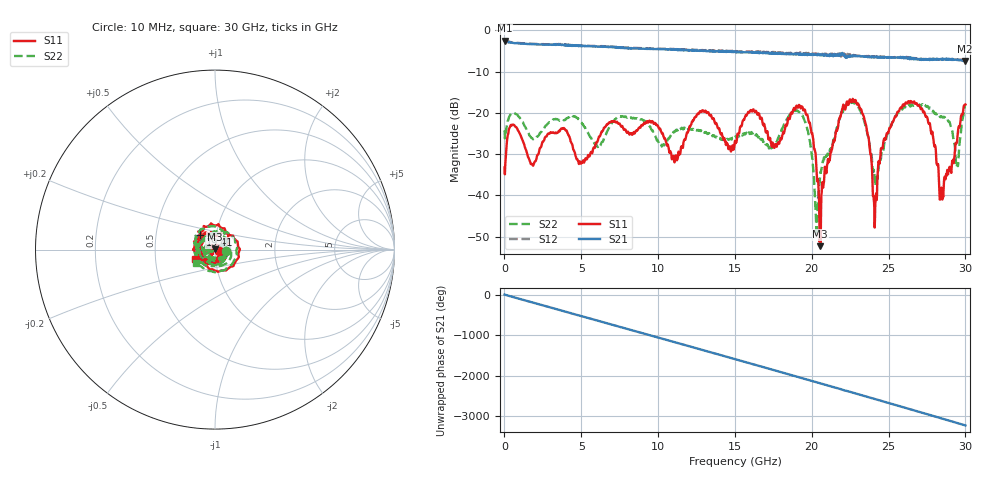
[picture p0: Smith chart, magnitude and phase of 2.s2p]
!Agilent Technologies,E8364B,US42250130,A.04.87.01
!Agilent E8364B: A.04.87.01
!Date: Monday, February 07, 2022 23:47:05
!Correction: S11(Full 2 Port SOLT,1,2) S21(Full 2 Port SOLT,1,2) S12(Full 2 Port SOLT,1,2) S22(Full 2 Port SOLT,1,2)
!S2P File: Measurements: S11, S21, S12, S22:
# Hz S  dB  R 50
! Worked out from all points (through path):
!   1601 points, 10 MHz to 30 GHz, reference 50 ohm
!   highest |S21| = -2.56 dB at 28.74 MHz (marker M1); lowest = -7.4 dB at 29.94 GHz (marker M2)
!   group delay of S21, straight-line fit = 298 ps
!   lowest |S11| = -52.3 dB at 20.55 GHz (marker M3), VSWR 1.00, Z = 49.9 + j0.212 ohm
!   |S11| at or under -10 dB: start of sweep to end of sweep
!   |S22| runs from -50.0 to -17.2 dB; largest |S21 - S12| = 0.069
!   S11 on the Smith chart (normalised r, x): 10 MHz: 1.04, -0.01; 19.41 GHz: 0.84, +0.14; 30 GHz: 0.79, -0.09
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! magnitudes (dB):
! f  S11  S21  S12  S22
! 10 MHz  -33.2  -2.6  -2.6  -24.2
! 28.74 MHz  -34.9  -2.6  -2.5  -26.2
! 534.8 MHz  -22.9  -3.0  -2.9  -20.1
! 1.772 GHz  -32.4  -3.4  -3.3  -26.1
! 3.796 GHz  -23.7  -3.6  -3.4  -22.0
! 5.015 GHz  -32.2  -3.8  -3.7  -22.3
! 10.02 GHz  -23.5  -4.6  -4.4  -27.0
! 11.13 GHz  -31.1  -4.7  -4.6  -24.5
! 15.01 GHz  -26.8  -5.2  -5.2  -26.0
! 19.41 GHz  -18.7  -5.9  -5.4  -20.7
! 20.01 GHz  -24.9  -5.8  -5.7  -30.2
! 20.31 GHz  -34.2  -5.9  -5.7  -50.0
! 20.55 GHz  -52.3  -5.8  -5.7  -34.8
! 22.17 GHz  -19.2  -6.4  -5.9  -18.2
! 23.36 GHz  -20.7  -6.3  -6.2  -21.4
! 24.11 GHz  -45.8  -6.4  -6.4  -37.2
! 25.01 GHz  -24.4  -6.7  -6.6  -24.5
! 27.08 GHz  -18.9  -6.9  -7.0  -18.2
! 28.44 GHz  -38.1  -6.9  -7.1  -20.8
! 29.46 GHz  -27.1  -7.2  -7.1  -32.5
! 29.94 GHz  -18.1  -7.4  -7.3  -18.7
! 30 GHz  -18.0  -7.3  -7.3  -17.9
